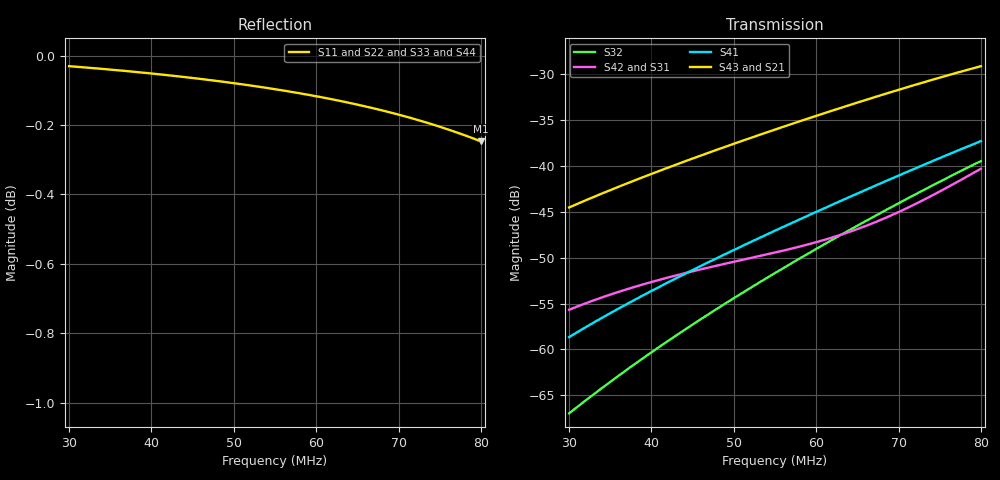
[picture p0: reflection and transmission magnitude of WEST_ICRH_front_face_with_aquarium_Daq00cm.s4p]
! Touchstone file exported from HFSS 2020.2.0
!  File:  C:/Users/JH218595/Documents/ICRH/WEST/HFSS_antenna_front_face/WEST_ICRH_front_face_with_aquarium.aedt
!  Generated:  11:46:09  oct. 12, 2020
!  Design:  with_aquarium
!  Project:  WEST_ICRH_front_face_with_aquarium
!  Setup:  Setup1
!  Solution:  Sweep
! Variables:
!  $epsr_water = 76.5 - 306i
!  AngMax = 180deg
!  B = 350mm
!  Daq = 0cm
!  Deemb = 150mm
!  Dint = 102mm
!  Dout = 222mm
!  H = 900mm
!  L = 900mm
!  P1 = 51mm
!  alpha0 = 160deg
!  beta0 = 10deg
!  eglass = 19mm
!  x0acq = -15mm
!  xs1 = -15mm
!  xs2 = 64.3471413188093mm
!  xs3 = 115.347141318809mm
!  xs4 = 115.347141318809mm
!  xs5 = 64.3471413188093mm
!  xsp1 = -34.2931056258292mm
!  xsp2 = 48.4042483264409mm
!  xsp3 = 134.347141318809mm
!  xsp4 = 134.347141318809mm
!  xsp5 = 48.4042483264409mm
!  xspp1 = -34.2931056258292mm
!  xspp2 = -34.2931056258292mm
!  xspp3 = 134.347141318809mm
!  xspp4 = 315.706894374171mm
!  xspp5 = 315.706894374171mm
!  ys2 = 450mm
!  ys3 = 450mm
!  ys4 = -450mm
!  ys5 = -450mm
!  ysp2 = 469mm
!  ysp3 = 469mm
!  ysp4 = -469mm
!  ysp5 = -469mm
!  yspp1 = -469mm
!  yspp2 = 469mm
!  yspp3 = 469mm
!  yspp4 = -450mm
!  yspp5 = -469mm
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# GHZ S MA
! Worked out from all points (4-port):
!   5001 points, 30 MHz to 80 MHz, reference per port
!   strongest paths, dB at 30 MHz, 42.5 MHz, 55 MHz, 67.5 MHz, 80 MHz:
!     S43: -44.5, -40.0, -36.0, -32.4, -29.1
!     S21: -44.5, -40.0, -36.1, -32.4, -29.2
!     S41: -58.7, -52.5, -47.1, -42.0, -37.3
!     S42: -55.7, -52.0, -49.4, -46.0, -40.3
!     S31: -55.7, -52.1, -49.5, -46.0, -40.3
!     S32: -67.0, -58.8, -51.7, -45.3, -39.5
!   lowest |S11| = -0.2 dB at 80 MHz (marker M1), VSWR 70.33
!   |S11| at or under -10 dB: nowhere
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0.03  0.9965 145.6  0.005932 63.3  0.001643 83.4  0.001167 -107.7
      0.005932 63.3  0.9965 145.5  0.0004484 -120.4  0.001645 83.4
      0.001643 83.4  0.0004484 -120.4  0.9965 145.5  0.005937 63.3
      0.001167 -107.7  0.001645 83.4  0.005937 63.3  0.9965 145.6
0.04437  0.9928 127.3  0.0107 45.5  0.002619 72.9  0.002622 -134.5
         0.0107 45.5  0.9928 127.1  0.001309 -148.5  0.002623 72.8
         0.002619 72.9  0.001309 -148.5  0.9928 127.1  0.01071 45.4
         0.002622 -134.5  0.002623 72.8  0.01071 45.4  0.9928 127.3
0.05877  0.9872 106.8  0.01794 22.7  0.003706 70.4  0.0053 -166.4
         0.01794 22.7  0.9873 106.5  0.003278 179.3  0.003709 70.3
         0.003706 70.4  0.003278 179.3  0.9872 106.5  0.01797 22.5
         0.0053 -166.4  0.003709 70.3  0.01797 22.5  0.9872 106.8
0.0645  0.9842 97.8  0.02173 12.0  0.004443 72.4  0.006909 179.5
        0.02173 12.0  0.9842 97.6  0.004588 165.3  0.004443 72.2
        0.004443 72.4  0.004588 165.3  0.9842 97.6  0.02177 11.9
        0.006909 179.5  0.004443 72.2  0.02177 11.9  0.9841 97.8
0.06986  0.9807 88.9  0.0258 1.1  0.005569 74.1  0.0088 165.4
         0.0258 1.1  0.9808 88.7  0.006206 151.4  0.005564 74.0
         0.005569 74.1  0.006206 151.4  0.9807 88.7  0.02586 0.9
         0.0088 165.4  0.005564 74.0  0.02586 0.9  0.9806 88.9
0.07494  0.9768 80.1  0.03014 -10.1  0.007239 73.8  0.011 151.2
         0.03014 -10.1  0.9769 79.8  0.008173 137.5  0.007228 73.7
         0.007239 73.8  0.008173 137.5  0.9767 79.8  0.03021 -10.3
         0.011 151.2  0.007228 73.7  0.03021 -10.3  0.9766 80.0
0.08  0.972 70.8  0.03487 -22.1  0.009664 70.5  0.01365 136.0
      0.03487 -22.1  0.9722 70.6  0.01062 122.6  0.009647 70.4
      0.009664 70.5  0.01062 122.6  0.972 70.6  0.03495 -22.4
      0.01365 136.0  0.009647 70.4  0.03495 -22.4  0.9718 70.8
